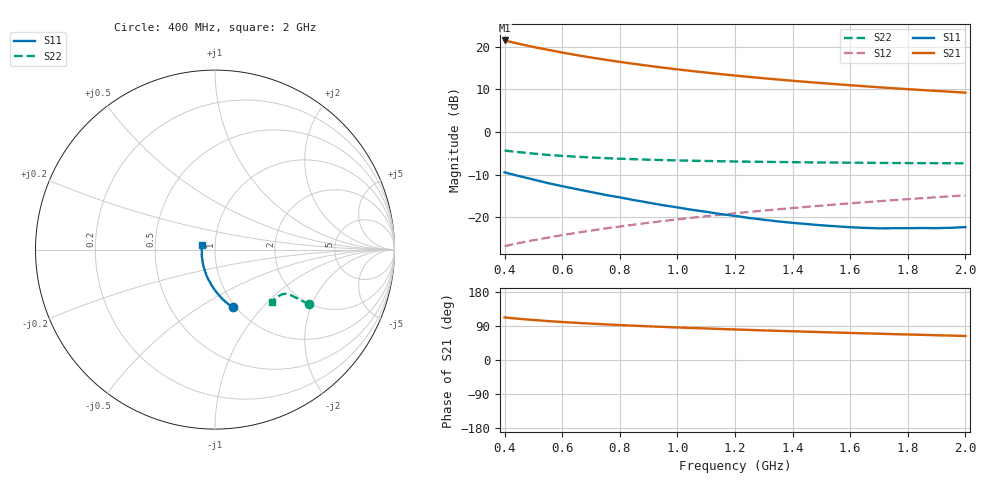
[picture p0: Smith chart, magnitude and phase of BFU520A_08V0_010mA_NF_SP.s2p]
! Filename:  P:\Prog\Test\Noise\ATS_data\Testdata_Net\06 Compressed Noise after Statistics\BFU520A_APG2013_30_A05_08p0V_010mA_NF_CM01_D.sf
! Date/Time: Wed 24/Apr/2013 20:06:20
! BFU520A_APG2013_30_A05_08p0V_1to20mA_NF_CM01_Bias6_R.sf
! Noise Parameter Data File
! BFU520A_APG2013_30_A05_08p0V_1to20mA_NF_CM01
! Date/time: Thu Apr 11 09:33:54 2013
! VAR V_out= 8.000000
! VAR I_out= 9.995000
! VAR V_in= 0.829900
! VAR I_in= 0.107105
! Device data file deembeded for feedlines and parallel
! Original file: \06 Compressed Noise after Statistics\BFU520A_APG2013_30_A05_08p0V_010mA_NF_CM01_R.sf
! Feed-files: PR017V01_150413_Feed1.s2p, PR017V01_150413_Feed2.s2p
! Parallel-file: PR017V01_150413_Par.s2p
# MHz S MA R 50
!  Freq-MHz  S11-mag  S11-arg  S21-mag  S21-arg  S12-mag  S12-arg  S22-mag  S22-arg
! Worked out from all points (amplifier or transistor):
!   37 points, 400 MHz to 2 GHz, reference 50 ohm
!   highest |S21| = 21.5 dB at 400 MHz (marker M1)
!   |S21| within 3 dB of that: start of sweep to 613.5 MHz
!   unconditionally stable (mu >= 1): 1.32 GHz to end of sweep
!   at 500 MHz: K = 0.82, MSG = 22.7 dB, |S12| = -25.4 dB
!   at 1.1 GHz: K = 0.98, MSG = 16.9 dB, |S12| = -19.8 dB
!   at 2 GHz: K = 1.00, MAG = 11.6 dB, |S12| = -14.9 dB
!   lowest NFmin = 0.84 dB at 433 MHz
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400  0.3358 -73.0  11.89 112.3  0.04566 68.8  0.6063 -30.0
420  0.3226 -74.8  11.46 110.8  0.0473 68.9  0.5949 -30.2
440  0.3099 -76.7  11.06 109.4  0.04889 68.9  0.5849 -30.3
460  0.2985 -78.3  10.67 108.1  0.05048 69.0  0.5756 -30.4
480  0.2875 -80.1  10.31 106.8  0.05207 69.1  0.5661 -30.5
500  0.2765 -81.7  9.978 105.6  0.05364 69.2  0.5583 -30.6
550  0.2515 -85.6  9.244 102.7  0.05753 69.5  0.5391 -30.6
600  0.2312 -89.2  8.575 100.3  0.06152 69.7  0.525 -30.7
650  0.2135 -92.6  8.006 98.1  0.06554 70.0  0.5127 -30.9
700  0.1974 -95.9  7.503 96.0  0.06958 70.2  0.5024 -30.9
750  0.1825 -99.1  7.055 94.0  0.07364 70.5  0.4934 -31.0
800  0.1709 -102.6  6.663 92.2  0.07773 70.7  0.4859 -31.2
850  0.1586 -105.9  6.309 90.5  0.08182 70.8  0.4791 -31.4
950  0.1382 -112.5  5.701 87.4  0.09004 71.0  0.4684 -31.8
1050  0.1221 -119.4  5.202 84.5  0.09836 71.1  0.4601 -32.4
1150  0.1088 -127.1  4.787 81.8  0.1068 71.1  0.4535 -33.1
1200  0.1035 -130.6  4.605 80.6  0.1111 71.0  0.4508 -33.5
1350  0.08915 -142.9  4.132 76.9  0.1238 70.8  0.4444 -34.8
1500  0.08026 -156.6  3.755 73.6  0.1367 70.4  0.4386 -36.3
1650  0.07492 -170.0  3.446 70.3  0.1498 69.8  0.4354 -38.1
1750  0.07422 -179.3  3.266 68.3  0.1584 69.4  0.4324 -39.3
2000  0.07645 160.7  2.903 63.4  0.1804 68.3  0.4287 -42.7
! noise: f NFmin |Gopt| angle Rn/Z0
400  0.8772  0.02164  -6.83  0.1174
460  0.8479  0.02676  -164.2  0.1019
600  0.9389  0.02883  -41.88  0.1328
800  0.905  0.03268  -175.5  0.1031
1000  0.9419  0.05742  -170.5  0.0976
1200  0.9804  0.06536  -159.8  0.1
1400  1.03  0.08164  -143.9  0.0959
1600  1.034  0.09889  -162.4  0.0903
1800  0.997  0.1489  -163.7  0.0818
2000  0.9968  0.1784  -144.3  0.0884
